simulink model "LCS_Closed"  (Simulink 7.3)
settings: Solver=ode45  StartTime=0.0  StopTime=50  RelTol=1e-3
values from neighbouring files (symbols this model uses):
  d2r = pi/180    (= 0.0174532925199)    [run.m]
  kls = [0.23009875115  -1.3857134134    0.5565800989    0.03843893525  0.1360972015;        0.22658853965   0.3268097242   -0.0904376422    0.0272194403  -0.00768778705]    [run.m]
  r2d = 180/pi    (= 57.2957795131)    [Pl.m]    (also in run.m)
undefined symbols (not defined in the file or in its folder): Alv, Blv, Clv, Dlv, KSmix

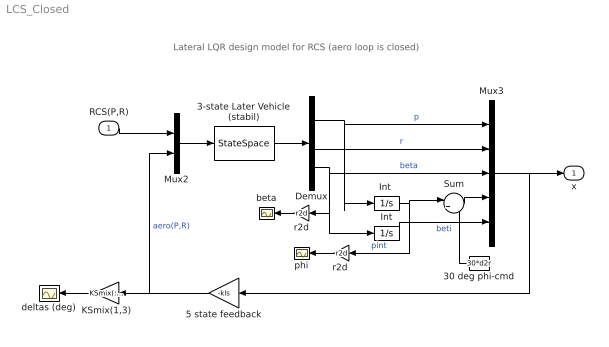
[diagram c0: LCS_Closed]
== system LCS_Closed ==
  note: Lateral LQR design model for RCS (aero loop is closed)
  RCS(P,R) : Inport  OutDataType=sfix(16)  OutScaling=2^0
  3-state Later Vehicle (stabil) : StateSpace  A=Alv  B=Blv  C=Clv  D=Dlv
  30 deg phi-cmd : Constant  Value=30*d2r  OutDataType=sfix(16)  OutScaling=2^0
  5 state feedback : Gain  Gain=-kls  Multiplication=Matrix(K*u)  ParameterDataType=sfix(16)  ParameterScaling=2^0  OutDataType=sfix(16)  OutScaling=2^0
  Demux : Demux  Outputs=3
  Int : Integrator
  "Int " : Integrator
  KSmix(1,3) : Gain  Gain=KSmix(:,[1,3])*r2d  Multiplication=Matrix(K*u)  ParameterDataType=sfix(16)  ParameterScaling=2^0  OutDataType=sfix(16)  OutScaling=2^0
  Mux2 : Mux  Inputs=[2,2]
  Mux3 : Mux  Inputs=5
  Sum : Sum  Inputs=|+-  OutDataType=sfix(16)  OutScaling=2^0
  beta : Scope
  deltas (deg) : Scope
  phi : Scope
  r2d : Gain  Gain=r2d  ParameterDataType=sfix(16)  ParameterScaling=2^0  OutDataType=sfix(16)  OutScaling=2^0
  "r2d " : Gain  Gain=r2d  ParameterDataType=sfix(16)  ParameterScaling=2^0  OutDataType=sfix(16)  OutScaling=2^0
  x : Outport  OutDataType=sfix(16)  OutScaling=2^0
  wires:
  3-state Later Vehicle (stabil)/1 -> Demux/1
  Demux/1 -> Mux3/1, "Int "/1  "p"
  Demux/2 -> Mux3/2  "r"
  Mux2/1 -> 3-state Later Vehicle (stabil)/1
  RCS(P,R)/1 -> Mux2/1
  Demux/3 -> Mux3/3, r2d/1, Int/1  "beta"
  5 state feedback/1 -> Mux2/2, KSmix(1,3)/1  "aero(P,R)"
  KSmix(1,3)/1 -> deltas (deg)/1
  r2d/1 -> beta/1
  Mux3/1 -> x/1, 5 state feedback/1
  "Int "/1 -> Sum/1, "r2d "/1  "pint"
  30 deg phi-cmd/1 -> Sum/2
  Sum/1 -> Mux3/4
  Int/1 -> Mux3/5  "beti"
  "r2d "/1 -> phi/1
